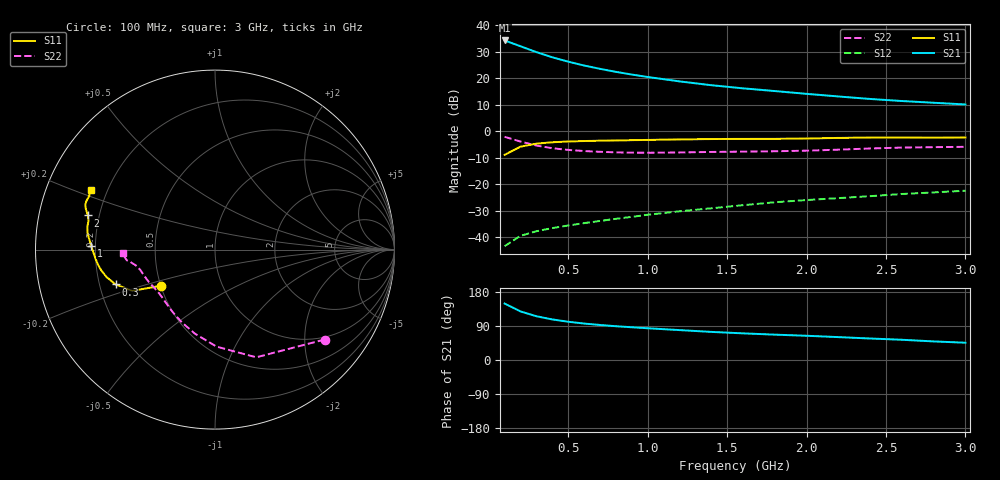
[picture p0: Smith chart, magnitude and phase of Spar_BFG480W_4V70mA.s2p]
! Filename: 470BFG480.001
! Title: BFG480W
! Bias: Vce=4V; Ic=70mA
! Company: NXP Semiconductors NL
! User: Quality&Reliability T&D
! Measure time: 10 Nov 1999 / 12:03:23
#  MHz  S  MA  R 50
! Freq  S11  S21  S12  S22  :
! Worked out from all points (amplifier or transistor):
!   20 points, 100 MHz to 3 GHz, reference 50 ohm
!   highest |S21| = 34.3 dB at 100 MHz (marker M1)
!   |S21| within 3 dB of that: start of sweep to 236.8 MHz
!   unconditionally stable (mu >= 1): 840 MHz to end of sweep
!   at 400 MHz: K = 0.73, MSG = 32.2 dB, |S12| = -36.5 dB
!   at 1.2 GHz: K = 1.06, MAG = 23.0 dB, |S12| = -30.2 dB
!   at 3 GHz: K = 1.05, MAG = 14.9 dB, |S12| = -22.4 dB
!   S11 on the Smith chart (normalised r, x): 100 MHz: 0.50, -0.23; 300 MHz: 0.27, -0.16; 1 GHz: 0.18, +0.02; 2 GHz: 0.16, +0.13; 3 GHz: 0.14, +0.22
100  0.3608 -146.1  51.95 148.9  0.006828 68.5  0.7902 -39.3
200  0.515 -153.5  40.41 128.2  0.0107 58.6  0.6426 -69.1
300  0.5869 -160.7  31.29 115.5  0.01307 56.1  0.5403 -89.2
400  0.6233 -165.8  25.01 107.1  0.01498 57.0  0.4816 -103.4
500  0.6445 -169.7  20.68 100.9  0.01676 58.8  0.4472 -113.9
600  0.6578 -172.8  17.5 96.2  0.01857 60.6  0.4259 -121.8
700  0.6669 -175.5  15.14 92.4  0.02043 62.9  0.4117 -128.0
800  0.6744 -177.8  13.29 89.2  0.0224 64.7  0.4022 -133.2
900  0.6829 -179.9  11.81 86.4  0.02438 66.7  0.3971 -137.7
1000  0.6901 178.1  10.63 83.8  0.02673 68.0  0.3953 -141.7
1200  0.7054 174.9  8.782 78.9  0.03102 70.2  0.4001 -148.2
1400  0.7168 172.4  7.439 74.2  0.03539 71.6  0.4094 -153.1
1600  0.7223 169.9  6.489 70.3  0.04051 72.8  0.4152 -156.8
1800  0.7228 167.3  5.77 66.9  0.04598 73.6  0.4218 -160.7
2000  0.7335 164.9  5.108 63.9  0.05062 74.4  0.4327 -165.2
2200  0.753 162.7  4.561 60.4  0.05506 74.7  0.4516 -169.0
2400  0.7649 160.9  4.09 56.7  0.0599 74.3  0.4759 -171.6
2600  0.766 159.3  3.74 53.4  0.0659 73.9  0.495 -173.1
2800  0.7618 157.0  3.471 49.0  0.07059 72.6  0.5039 -175.0
3000  0.7667 154.3  3.222 45.6  0.07599 72.0  0.5114 -177.9
